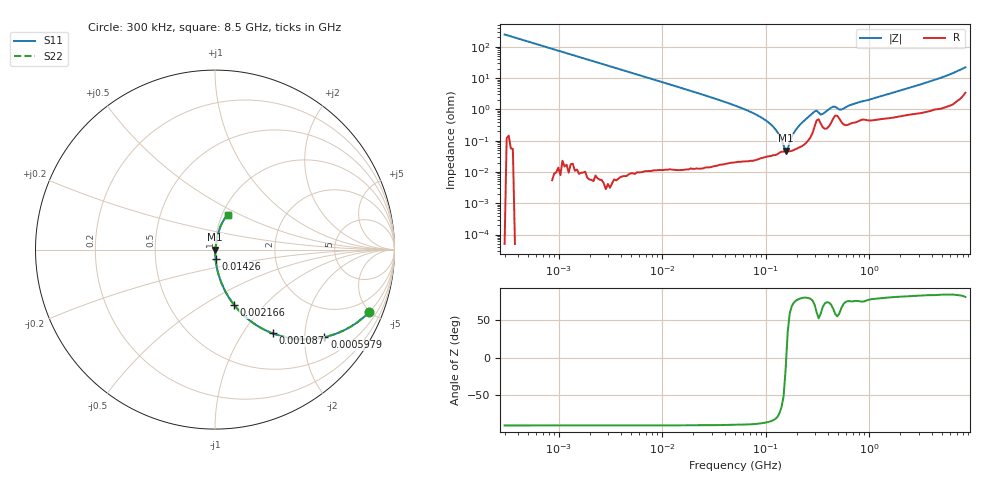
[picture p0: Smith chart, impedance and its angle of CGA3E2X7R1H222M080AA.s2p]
! S-parameter Generated by TDK Corporation
! Copyright(C) 2015 TDK Corporation.
! All Rights Reserved.
! TDK P/N: CGA3E2X7R1H222M080AA (Multilayer Ceramic Chip Capacitors)
! Property: C=2.2nF
! Size(LxWxT): 1.6x0.8x0.8mm, 0.063x0.031x0.031inches
! Model Type: s2p (Touchstone File Format Version 1.0)
! Frequency: DC=Yes Start=0.3MHz Stop=8500MHz 225points Log-sweep
! Note:
! Model Generated on Jun. 23, 2015
! Hash(MD5):
! Port Assignments:
!  1 ---| |--- 2
! Applicable Conditions:
!  Temperature = 25 degC
!  DC Bias Voltage = 0 V
!  Small Signal Operation
! Terms and conditions regarding TDK Simulation Models
! (1)This simulation model is being provided solely for informational purposes. Please refer to the specifications of the products in terms of detailed characteristics of such products.
! (2)In no event shall TDK Corporation of any of its subsidiaries be liable for any loss or damage arising, directly or indirectly,
!  From any information contained in this simulation model, including, but not limited to loss or damages arising from any inaccuracies, omissions or errors in connection with such information.
! (3)Any and all copyrights on this simulation model are owned by TDK Corporation.
!  Duplication or redistribution of this simulation model without prior written permission from TDK Corporation is prohibited.
! (4)This simulation model is subject to any modification or change without any prior notice.
! (5)Neither TDK Corporation nor any of its subsidiaries shall make any warranty, express or implied,
!  Including but not limited to the correctness, implied warranties of merchantability and fitness for a particular purpose with respect to this simulation models.
! (6)The use of this simulation model shall be deemed to have consented to the terms and conditions hereof.
# MHz S MA R 50
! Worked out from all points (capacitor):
!   224 points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, 300 kHz to 8.5 GHz, reference 50 ohm
!   read as one part in series: C = 2.14 nF near 314.1 kHz
!   lowest |Z| = 47.5 mohm at 155.7 MHz (marker M1)
!   series resonance near 157.9 MHz, so ESL is about 480 pH
!   S11 on the Smith chart (normalised r, x): 300 kHz: 1.00, -4.96; 597.9 kHz: 1.00, -2.50; 1.087 MHz: 1.00, -1.37; 2.166 MHz: 1.00, -0.69; 14.26 MHz: 1.00, -0.10; 8.5 GHz: 1.07, +0.44
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0.3  0.9275 -21.9  0.3737 68.1  0.3737 68.1  0.9275 -21.9
0.597865  0.7806 -38.7  0.6251 51.3  0.6251 51.3  0.7806 -38.7
1.086811  0.5662 -55.5  0.8241 34.5  0.8241 34.5  0.5662 -55.5
1.72111  0.398 -66.5  0.9173 23.5  0.9173 23.5  0.398 -66.5
2.165888  0.326 -71.0  0.9453 19.0  0.9453 19.0  0.326 -71.0
9.430415  0.07871 -85.4  0.9968 4.5  0.9968 4.5  0.07871 -85.4
14.2633  0.05189 -86.9  0.9985 3.0  0.9985 3.0  0.05189 -86.9
51.67171  0.0129 -88.4  0.9997 0.7  0.9997 0.7  0.0129 -88.4
81.82903  0.006665 -87.5  0.9997 0.4  0.9997 0.4  0.006665 -87.5
112.8926  0.003235 -84.1  0.9997 0.2  0.9997 0.2  0.003235 -84.1
135.6836  0.001464 -73.7  0.9996 0.1  0.9996 0.1  0.001464 -73.7
155.7485  0.0004737 -15.1  0.9995 0.0  0.9995 0.0  0.0004737 -15.1
163.0757  0.0005458 33.9  0.9995 -0.0  0.9995 -0.0  0.0005458 33.9
178.7805  0.001321 68.9  0.9995 -0.1  0.9995 -0.1  0.001321 68.9
195.9978  0.002258 76.0  0.9995 -0.1  0.9995 -0.1  0.002258 76.0
283.1228  0.007468 76.0  0.9982 -0.4  0.9982 -0.4  0.007468 76.0
310.3886  0.009045 60.2  0.9955 -0.5  0.9955 -0.5  0.009045 60.2
340.2802  0.006798 58.8  0.9965 -0.3  0.9965 -0.3  0.006798 58.8
448.3627  0.01217 65.0  0.9949 -0.6  0.9949 -0.6  0.01217 65.0
538.8791  0.009872 66.0  0.996 -0.5  0.996 -0.5  0.009872 66.0
1551.304  0.03123 78.6  0.9943 -1.8  0.9943 -1.8  0.03123 78.6
8500  0.2091 69.2  0.946 -11.9  0.946 -11.9  0.2091 69.2
